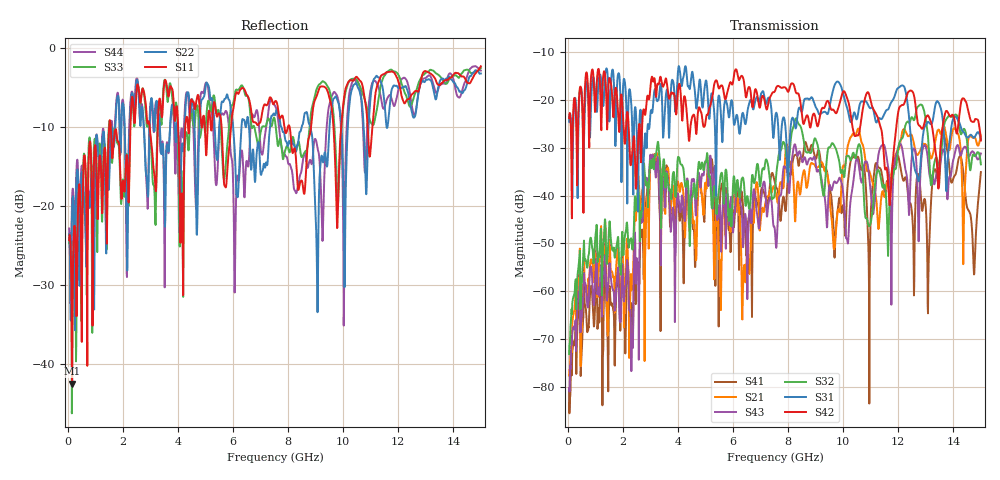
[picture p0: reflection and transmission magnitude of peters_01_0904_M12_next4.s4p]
# MHZ S RI R 50.00
! FREQ  S11  S12  S13  S14
!  S21  S22  S23  S24
!  S31  S32  S33  S34
!  S41  S42  S43  S44
!  REAL  IMAG  REAL  IMAG  REAL  IMAG  REAL  IMAG
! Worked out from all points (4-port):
!   1496 points, 50 MHz to 15 GHz, reference 50 ohm
!   strongest paths, dB at 50 MHz, 3.79 GHz, 7.53 GHz, 11.27 GHz, 15 GHz:
!     S42: -23.8, -18.5, -18.0, -23.8, -28.5
!     S31: -24.5, -15.7, -23.7, -24.0, -28.2
!     S32: -73.2, -37.6, -38.6, -34.6, -33.4
!     S43: -80.3, -45.1, -47.9, -31.8, -31.2
!     S21: -77.7, -38.5, -39.0, -46.6, -27.4
!     S41: -80.9, -39.6, -37.5, -34.0, -35.1
!   lowest |S11| = -42.5 dB at 160 MHz (marker M1), VSWR 1.02, Z = 49.7 + j0.69 ohm
!   |S11| at or under -10 dB: start of sweep to 1.505 GHz; 1.561 GHz to 2.275 GHz (713.7 MHz wide, 37.2 % of centre); 8.057 GHz to 8.833 GHz (775.9 MHz wide, 9.19 % of centre)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
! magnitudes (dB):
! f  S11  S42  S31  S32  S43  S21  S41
! 50 MHz  -24.3  -23.8  -24.5  -73.2  -80.3  -77.7  -80.9
! 160 MHz  -42.5  -34.0  -40.7  -63.2  -69.3  -67.2  -73.7
! 2.31 GHz  -7.0  -32.9  -21.1  -49.1  -76.8  -56.7  -63.0
! 3.09 GHz  -14.1  -15.9  -21.6  -32.3  -31.7  -31.5  -31.6
! 6.39 GHz  -5.1  -15.9  -23.3  -37.0  -47.7  -55.2  -44.3
! 7.95 GHz  -10.6  -17.7  -30.2  -32.9  -34.4  -29.2  -40.0
! 15 GHz  -2.3  -28.5  -28.2  -33.4  -31.2  -27.4  -35.1
